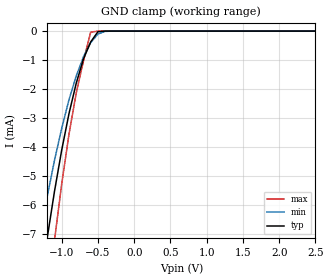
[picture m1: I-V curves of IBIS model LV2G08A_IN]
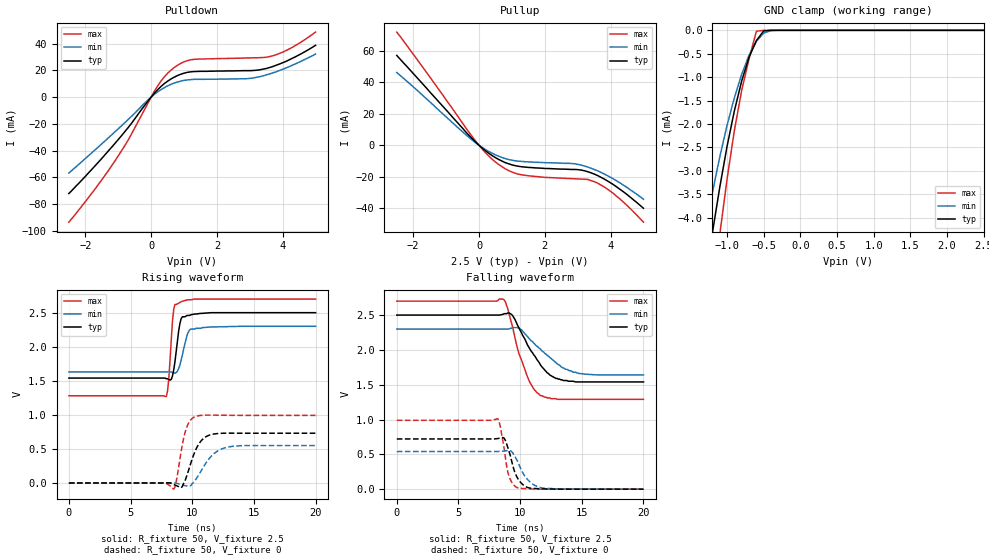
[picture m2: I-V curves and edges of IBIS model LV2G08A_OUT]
|/_/_/_/_/_/_/_/_/_/_/_/_/_/_/_/_/_/_/_/_/_/_/_/_/_/_/_/_/_/_/_/_/_/_/_/_/_/
|   Renesas Electronics Corp.
|   Multi Purpose Semiconductor Digital IC Design Group
|   IBIS Model of HD74LV2G08A
|   2.5V Dual 2-input AND Gates,  SSOP-8(8pin) Package
|   History
|   V1.0   April   1, 2003   : First release.
|/_/_/_/_/_/_/_/_/_/_/_/_/_/_/_/_/_/_/_/_/_/_/_/_/_/_/_/_/_/_/_/_/_/_/_/_/_/
[IBIS Ver]   2.1
[Comment Char]  |_char
[File name]   l2g08s2.ibs
[File Rev]   1.1
[Date]   April 1, 2003
[Source]   Data created from SPICE simulations at
|   Renesas Electronics Corp.
[Notes]   RLC value of the Package is determined by assuming typical
|   conditions.
[Disclaimer]   This information is for modeling purposes only, and is not
|   guaranteed.
[Copyright]   Copyright 2003, Renesas Electronics Corp.,
|   All Rights Reserved.
|   Component  HD74LV2G08A
[Component]   HD74LV2G08A
[Manufacturer]  Renesas Electronics Corp.
[Package]
|   typ   min   max
R_pkg   0.099   0.095   0.102
L_pkg   1.740nH   1.680nH   1.790nH
C_pkg   0.140pF   0.140pF   0.150pF
[Pin]   signal_name   model_name   R_pin   L_pin   C_pin
1   1A   LV2G08A_IN   0.102   1.780nH   0.140pF
2   1B   LV2G08A_IN   0.097   1.710nH   0.150pF
3   2Y   LV2G08A_OUT   0.095   1.680nH   0.150pF
4   GND   GND   0.102   1.790nH   0.140pF
5   2A   LV2G08A_IN   0.101   1.790nH   0.140pF
6   2B   LV2G08A_IN   0.097   1.710nH   0.150pF
7   1Y   LV2G08A_OUT   0.097   1.710nH   0.150pF
8   VCC   POWER   0.102   1.790nH   0.140pF
| Models and submodels in the file (2): LV2G08A_IN (Input), LV2G08A_OUT (Output)
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|   Model  LV2G08A_IN
[Model]   LV2G08A_IN
Model_type  Input
Vinl = 0.75V
Vinh = 1.75V
| variable   typ   min   max
C_comp   2.35pF   2.25pF   2.45pF
| variable   typ   min   max
[Temperature range]   25   85   -40
| variable   typ   min   max
[Voltage range]   2.5V   2.3V   2.7V
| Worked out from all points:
|   GND clamp passes 1 mA (typ) near -0.70 V on its own axis
[GND Clamp]
|   Voltage   I(typ)   I(min)   I(max)
-2.5V     -38.3mA    -30.7mA    -49.7mA
-1.3V     -8.88mA    -7.07mA    -11.7mA
-1.2V     -7.13mA    -5.7mA     -9.39mA
-1.1V     -5.53mA    -4.46mA    -7.22mA
-1V       -4.1mA     -3.35mA    -5.27mA
-900mV    -2.85mA    -2.37mA    -3.56mA
-800mV    -1.8mA     -1.55mA    -2.14mA
-700mV    -962uA     -887uA     -1.03mA
-600mV    -372uA     -399uA     -36.9uA
-500mV    -22uA      -101uA     -445nA
-400mV    -433nA     -10.3uA    -2.54nA
2.5V      5.09pA     27.7pA     5pA
|   Model  LV2G08A_OUT
[Model]   LV2G08A_OUT
Model_type  Output
Polarity   Inverting
Vmeas = 1.25V
| variable   typ   min   max
C_comp   4.85pF   4.75pF   4.95pF
| variable   typ   min   max
[Temperature range]   25   85   -40
| variable   typ   min   max
[Voltage range]   2.5V   2.3V   2.7V
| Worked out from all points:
|   slope of the pulldown table from 0 to 0.375 V, typ, clamps not added: 39.2 ohm
|   slope of the pullup table from 0 to 0.375 V, typ, clamps not added: 60.8 ohm
|   GND clamp passes 1 mA (typ) near -0.78 V on its own axis
|   rising waveform, R_fixture 50, V_fixture 2.5: 20-80 % time 411ps typ, 531ps min, 309ps max; typ from 1.54 V to 2.5 V
|   rising waveform, R_fixture 50, V_fixture 0: 20-80 % time 946ps typ, 1.33ns min, 634ps max; typ from 0 V to 0.73 V
|   falling waveform, R_fixture 50, V_fixture 2.5: 20-80 % time 1.96ns typ, 2.53ns min, 1.44ns max; typ from 2.5 V to 1.54 V
|   falling waveform, R_fixture 50, V_fixture 0: 20-80 % time 804ps typ, 1.08ns min, 580ps max; typ from 0.721 V to 0 V
[Pullup]
|   Voltage   I(typ)   I(min)   I(max)
-2.5V     56.9mA     46.1mA     71.7mA
-200mV    4.01mA     3.18mA     5.31mA
200mV     -3.53mA    -2.75mA    -4.76mA
500mV     -7.83mA    -6.06mA    -10.6mA
900mV     -11.7mA    -8.98mA    -16mA
1.2V      -13.3mA    -10.1mA    -18.3mA
2.9V      -15.3mA    -11.7mA    -21.2mA
3.3V      -16.7mA    -13.7mA    -21.6mA
3.5V      -18.2mA    -15.3mA    -23mA
4.1V      -25.1mA    -21.5mA    -30.8mA
4.5V      -31.2mA    -26.7mA    -38.1mA
5V        -39.9mA    -34.2mA    -48.7mA
[Pulldown]
|   Voltage   I(typ)   I(min)   I(max)
-2.5V     -72mA      -56.7mA    -93.4mA
-1.7V     -51.2mA    -39.3mA    -68.5mA
-1.1V     -34.6mA    -25.9mA    -47.7mA
-700mV    -22.8mA    -16.8mA    -32.2mA
200mV     5.59mA     3.93mA     8.44mA
700mV     14.9mA     10.5mA     22.1mA
1V        17.9mA     12.5mA     26.4mA
1.3V      19.1mA     13.3mA     28.2mA
2.9V      19.8mA     13.8mA     29.3mA
3.7V      22.9mA     18.1mA     30.9mA
4.3V      29.1mA     23.9mA     37.3mA
5V        38.7mA     32.2mA     48.6mA
[GND Clamp]
|   Voltage   I(typ)   I(min)   I(max)
-2.5V     -23.4mA    -18.8mA    -30.3mA
-1.3V     -5.4mA     -4.31mA    -7.13mA
-1.2V     -4.33mA    -3.47mA    -5.69mA
-1.1V     -3.36mA    -2.71mA    -4.37mA
-1V       -2.48mA    -2.03mA    -3.18mA
-900mV    -1.72mA    -1.44mA    -2.14mA
-800mV    -1.08mA    -936uA     -1.28mA
-700mV    -575uA     -533uA     -610uA
-600mV    -219uA     -237uA     -20.5uA
-500mV    -12.9uA    -58.6uA    -245nA
-400mV    -248nA     -6.13uA    -1.4nA
2.5V      2.62pA     30.9pA     2.5pA
[Ramp]
| variable   typ   min   max
dV/dt_r   0.433/924.8p   0.325/1.299n   0.593/629.1p
dV/dt_f   0.578/1.955n   0.400/2.552n   0.847/1.442n
R_load = 50ohms
[Rising Waveform]
R_fixture = 50
V_fixture = 2.5
V_fixture_min = 2.3
V_fixture_max = 2.7
C_fixture = 0p
|   Time   V(typ)   V(min)   V(max)
0s        1.54V      1.63V      1.28V
7.9ns     1.53V      1.63V      1.27V
8.1ns     1.52V      1.63V      1.53V
8.4ns     1.57V      1.62V      2.38V
8.5ns     1.66V      1.62V      2.55V
8.9ns     2.23V      1.68V      2.64V
9.2ns     2.44V      1.88V      2.67V
9.6ns     2.46V      2.18V      2.69V
9.9ns     2.47V      2.26V      2.69V
20ns      2.5V       2.3V       2.7V
[Rising Waveform]
R_fixture = 50
V_fixture = 0
C_fixture = 0p
|   Time   V(typ)   V(min)   V(max)
0s        273pV      604nV      141pV
7.8ns     273pV      604nV      141pV
8.5ns     -21.6mV    1.66mV     -91.2mV
8.7ns     -37.8mV    -3.78mV    19.8mV
9.1ns     -70.4mV    -23.9mV    461mV
9.4ns     23mV       -38.3mV    729mV
10.2ns    451mV      28.7mV     970mV
11.1ns    677mV      289mV      996mV
12.6ns    730mV      513mV      994mV
20ns      730mV      549mV      992mV
[Falling Waveform]
R_fixture = 50
V_fixture = 2.5
V_fixture_min = 2.3
V_fixture_max = 2.7
C_fixture = 0p
|   Time   V(typ)   V(min)   V(max)
0s        2.5V       2.3V       2.7V
8.6ns     2.51V      2.3V       2.73V
9ns       2.53V      2.3V       2.59V
9.4ns     2.49V      2.32V      2.32V
9.9ns     2.32V      2.31V      1.95V
10.6ns    2.07V      2.19V      1.61V
11.6ns    1.8V       2.02V      1.35V
12.9ns    1.59V      1.82V      1.3V
14.3ns    1.55V      1.68V      1.29V
20ns      1.54V      1.64V      1.29V
[Falling Waveform]
R_fixture = 50
V_fixture = 0
C_fixture = 0p
|   Time   V(typ)   V(min)   V(max)
0s        721mV      540mV      989mV
8.2ns     727mV      541mV      1.01V
8.4ns     736mV      543mV      890mV
8.7ns     732mV      548mV      588mV
8.9ns     652mV      553mV      338mV
9.1ns     543mV      555mV      185mV
9.8ns     156mV      398mV      19.5mV
10.6ns    24.2mV     138mV      4.91mV
11.6ns    5.59mV     24.4mV     475uV
20ns      -60.2uV    -110uV     -20.8uV
